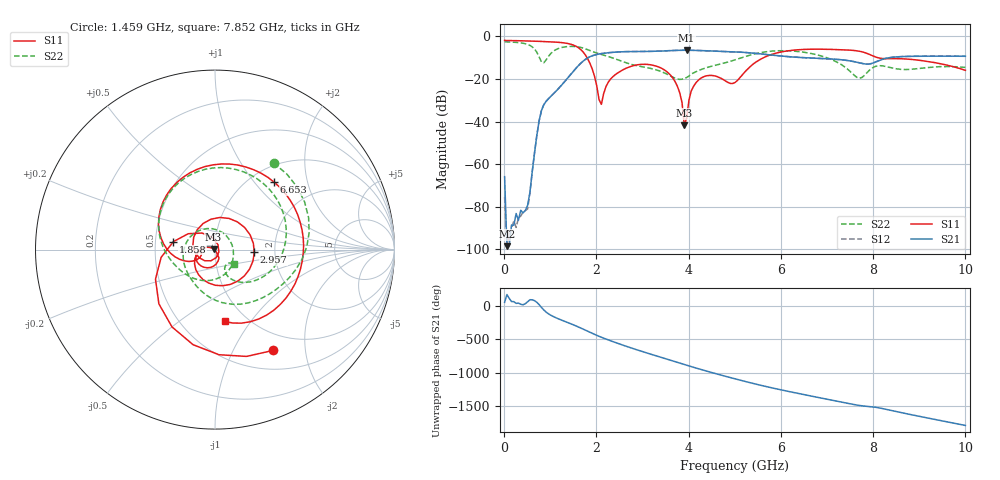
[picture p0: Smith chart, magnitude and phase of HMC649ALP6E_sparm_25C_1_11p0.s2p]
!Analog Devices Inc..
!GaAs MMIC 6-BIT DIGITAL PHASE SHIFTER, 3 - 6 GHz
!Filename: HMC649ALP6E_sparm_25C_1_11p0.s2p
!  :25C = 25degC
!  :_1_ = Sn1
!  :_11p0  = 11.0 state
!Device type:
!2 Port Calibration to sma connectors
!Phase Shifter:  0.000
!	Vss= -5V, Vdd= +5V , control Voltage = 0/ +5V
!Freq	S11	S11	S21	S21	S12	S12	S22	S22
! GHz	Mag dB	Degrees	Mag dB	Degrees	Mag dB	Degrees	Mag dB	Degrees
# GHZ S DB R 50.0
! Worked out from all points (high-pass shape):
!   201 points, 10 MHz to 10 GHz, reference 50 ohm
!   highest |S21| = -6.50 dB at 3.956 GHz (marker M1); lowest = -98.6 dB at 59.95 MHz (marker M2)
!   |S21| within 3 dB of the highest: 1.867 GHz to 6.151 GHz (4.285 GHz wide, 107 % of centre); 8.609 GHz to end of sweep
!   lowest |S11| = -41.7 dB at 3.906 GHz (marker M3), VSWR 1.02, Z = 49.2 + j0.296 ohm
!   |S11| at or under -10 dB: 1.797 GHz to 5.623 GHz (3.826 GHz wide, 103 % of centre); 8.099 GHz to end of sweep
!   |S22| runs from -20.2 to -2.5 dB; largest |S21 - S12| = 0.00069
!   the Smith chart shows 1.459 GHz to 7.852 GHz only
!   S11 on the Smith chart (normalised r, x): 1.459 GHz: 0.75, -1.45; 1.858 GHz: 0.62, +0.06; 2.957 GHz: 1.56, -0.05; 6.653 GHz: 1.27, +1.27; 7.852 GHz: 0.79, -0.76
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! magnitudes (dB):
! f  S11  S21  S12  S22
! 10 MHz  -1.9  -65.9  -75.6  -2.5
! 59.95 MHz  -1.9  -98.6  -97.5  -2.6
! 509.5 MHz  -2.1  -79.3  -81.1  -3.8
! 809.2 MHz  -2.4  -34.8  -34.8  -12.0
! 1.459 GHz  -3.8  -17.5  -17.5  -4.7
! 1.708 GHz  -7.2  -11.7  -11.7  -5.5
! 1.858 GHz  -12.5  -9.6  -9.6  -6.6
! 2.108 GHz  -31.9  -8.1  -8.1  -8.5
! 2.358 GHz  -18.9  -7.5  -7.5  -10.2
! 2.957 GHz  -13.2  -7.1  -7.1  -14.1
! 3.357 GHz  -14.4  -6.9  -6.9  -16.1
! 3.756 GHz  -23.4  -6.6  -6.6  -20.0
! 3.906 GHz  -41.7  -6.5  -6.5  -19.8
! 3.956 GHz  -38.4  -6.5  -6.5  -19.3
! 4.056 GHz  -25.6  -6.5  -6.5  -17.7
! 4.256 GHz  -19.8  -6.7  -6.6  -15.7
! 5.005 GHz  -21.7  -7.3  -7.3  -11.0
! 6.653 GHz  -6.0  -10.2  -10.2  -8.0
! 6.703 GHz  -6.0  -10.2  -10.2  -8.3
! 7.852 GHz  -7.9  -13.0  -13.0  -17.4
! 8.352 GHz  -10.5  -10.0  -10.0  -14.5
! 10 GHz  -16.0  -9.3  -9.3  -14.6
